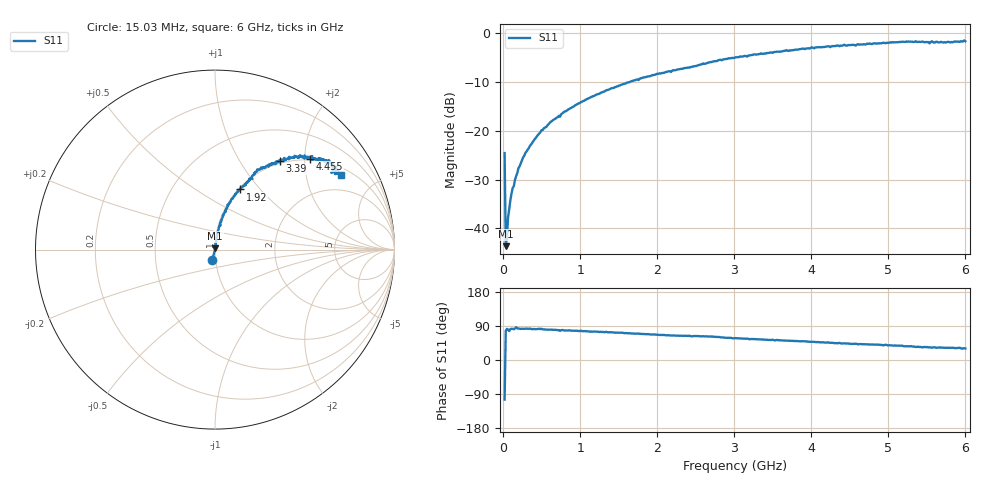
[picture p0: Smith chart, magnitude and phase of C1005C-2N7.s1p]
!	Network	Analyzer	HP8753E.07.74:	Oct	30	2002	Serial	No.	JP38451487
!	Hewlett-Packard
!	7	Sep	2009	8:21:07
!	Frequency	S11
#	HZ	S	RI	R	50
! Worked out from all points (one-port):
!   400 points, 15.03 MHz to 6 GHz, reference 50 ohm
!   lowest |S11| = -43.6 dB at 30.03 MHz (marker M1), VSWR 1.01, Z = 50.1 + j0.645 ohm
!   |S11| at or under -10 dB: start of sweep to 1.65 GHz
!   S11 on the Smith chart (normalised r, x): 15.03 MHz: 0.96, -0.11; 1.92 GHz: 1.02, +0.78; 3.39 GHz: 0.96, +1.52; 4.455 GHz: 0.97, +2.13; 6 GHz: 1.29, +3.18
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1.502992e7  -0.0147 -0.057
3.002985e7  0.00148 0.00643
4.502978e7  0.00111 0.00803
6.00297e7  0.00216 0.0129
9.002955e7  0.00274 0.0193
1.200294e8  0.00346 0.0257
1.350293e8  0.00419 0.0268
1.95029e8  0.00494 0.041
2.850286e8  0.00751 0.0587
4.950275e8  0.0135 0.1
7.650262e8  0.0278 0.147
1.095025e9  0.0526 0.205
1.515022e9  0.0894 0.275
1.92002e9  0.139 0.335
2.265019e9  0.181 0.379
3.015015e9  0.299 0.474
3.390013e9  0.363 0.494
3.765011e9  0.421 0.51
4.455008e9  0.531 0.507
4.515007e9  0.55 0.504
5.265004e9  0.657 0.475
5.445003e9  0.676 0.445
5.535002e9  0.647 0.429
5.565002e9  0.687 0.441
5.595002e9  0.656 0.438
5.625002e9  0.685 0.429
5.715001e9  0.666 0.427
6e9  0.702 0.414
